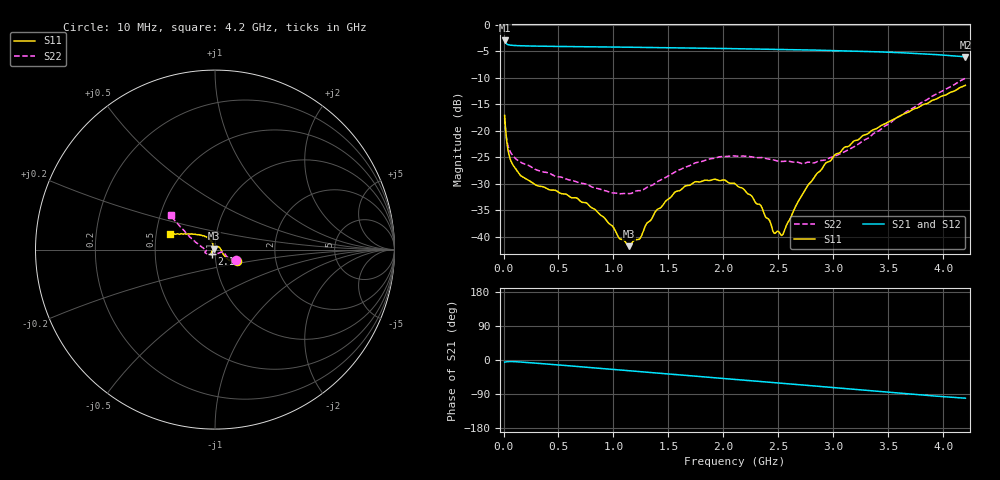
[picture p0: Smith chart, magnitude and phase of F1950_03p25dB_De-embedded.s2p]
! Integrated Device Technology
! Corporate Headquarters
! 6024 Silver Creek Valley Road
! San Jose, CA 95138  USA
! Phone:  1-408-284-8200
! Toll Free:  1-800-223-1366
! Webpage:  http://www.idt.com/
! Timing and RF Division
! 515 Groton Road, Suite 102
! Westford, MA 01886-6024
! Device:  F1950
! Description: 7-bit 0.25 dB Digital Step Attenuator
! Frequency:  150.0 -  4000.00 MHz
! Package:  4x4 mm Thin QFN Plastic Package: 24 pin
! Ports:  2 RF, 12 DC
!  Pin  1  = D0
!  Pin  2  = VDD
!  Pin  3  = Vmode
!  Pin  4  = GND
!  Pin  5  = RF1  =  Port 1
!  Pin  6  = GND
!  Pin  7  = GND
!  Pin  8  = GND
!  Pin  9  = GND
!  Pin 10  = GND
!  Pin 11  = GND
!  Pin 12  = GND
!  Pin 13  = GND
!  Pin 14  = RF2  =  Port 2
!  Pin 15  = GND
!  Pin 16  = LE
!  Pin 17  = CLK
!  Pin 18  = DATE
!  Pin 19  = D6
!  Pin 20  = D5
!  Pin 21  = D4
!  Pin 22  = D3
!  Pin 23  = D2
!  Pin 24  = D1
! State:  13
! Atten State:  3.25 dB
! Voltage:  +5.00 Volts
! Current:  Not Measured mA
! Data:  The device was measured on a the F195X evaluation board which has
!  individual transmission lines to the RF pins.  Data was collected
!  using a calibrated network analyzer.  The evaluation board was
!  de-embedded using a TRL calibration technique.
!  The reference plane is the edge of the package pin.
! Misc:  Board 2019
!  Action Tracker AT0250
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# GHz S dB R 50
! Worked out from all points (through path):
!   420 points, 10 MHz to 4.2 GHz, reference 50 ohm
!   highest |S21| = -2.99 dB at 10 MHz (marker M1); lowest = -6.1 dB at 4.2 GHz (marker M2)
!   group delay of S21, straight-line fit = 66.3 ps
!   lowest |S11| = -41.7 dB at 1.14 GHz (marker M3), VSWR 1.02, Z = 49.4 + j0.532 ohm
!   |S11| at or under -10 dB: start of sweep to end of sweep
!   |S22| runs from -31.9 to -10.1 dB; largest |S21 - S12| = 0.00078
!   S11 on the Smith chart (normalised r, x): 10 MHz: 1.27, -0.17; 2.11 GHz: 0.96, -0.05; 4.2 GHz: 0.59, +0.11
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0.01  -17.13 -28.2  -2.99 -5.7  -2.99 -5.7  -17.65 -27.0
0.04  -23.56 -34.5  -3.77 -4.3  -3.77 -4.3  -22.80 -29.4
0.06  -25.30 -30.0  -3.87 -4.0  -3.87 -4.0  -23.89 -25.5
0.16  -28.51 -12.0  -3.99 -5.4  -3.99 -5.4  -25.97 -19.6
0.71  -33.44 54.7  -4.16 -18.0  -4.16 -18.0  -29.89 -32.4
0.91  -36.27 77.5  -4.21 -22.7  -4.21 -22.8  -31.23 -49.5
1.14  -41.75 138.8  -4.26 -28.2  -4.26 -28.2  -31.85 -84.8
1.24  -40.34 176.9  -4.28 -30.5  -4.28 -30.5  -31.29 -100.2
1.3  -37.53 -164.8  -4.30 -32.0  -4.30 -32.0  -30.73 -110.7
1.41  -34.69 -149.4  -4.33 -34.6  -4.33 -34.6  -29.47 -124.7
1.56  -31.55 -139.4  -4.37 -38.1  -4.37 -38.1  -27.75 -138.9
1.74  -29.64 -131.9  -4.42 -42.4  -4.42 -42.5  -26.08 -150.6
1.92  -29.14 -128.0  -4.47 -46.7  -4.47 -46.8  -25.17 -158.8
2.11  -30.06 -126.6  -4.54 -51.3  -4.54 -51.3  -24.79 -164.1
2.34  -34.10 -137.4  -4.62 -56.8  -4.62 -56.8  -25.05 -168.5
2.46  -39.29 -167.0  -4.66 -59.6  -4.66 -59.6  -25.52 -169.7
2.53  -39.73 163.2  -4.68 -61.3  -4.68 -61.3  -25.79 -171.8
2.68  -33.32 119.3  -4.74 -64.9  -4.74 -65.0  -25.96 -173.4
2.81  -29.28 111.5  -4.80 -68.1  -4.79 -68.1  -26.06 -177.2
3.1  -23.13 118.4  -4.94 -75.3  -4.93 -75.3  -23.97 174.4
3.51  -18.23 137.3  -5.21 -85.3  -5.21 -85.4  -18.64 158.7
4.2  -11.44 160.7  -6.08 -100.7  -6.07 -100.8  -10.10 142.5
